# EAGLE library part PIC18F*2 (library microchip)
High-Performance, Enhanced Flash Microcontrollers with 10-Bit A/D Source: http://www.microchip.com .. 39564c.pdf
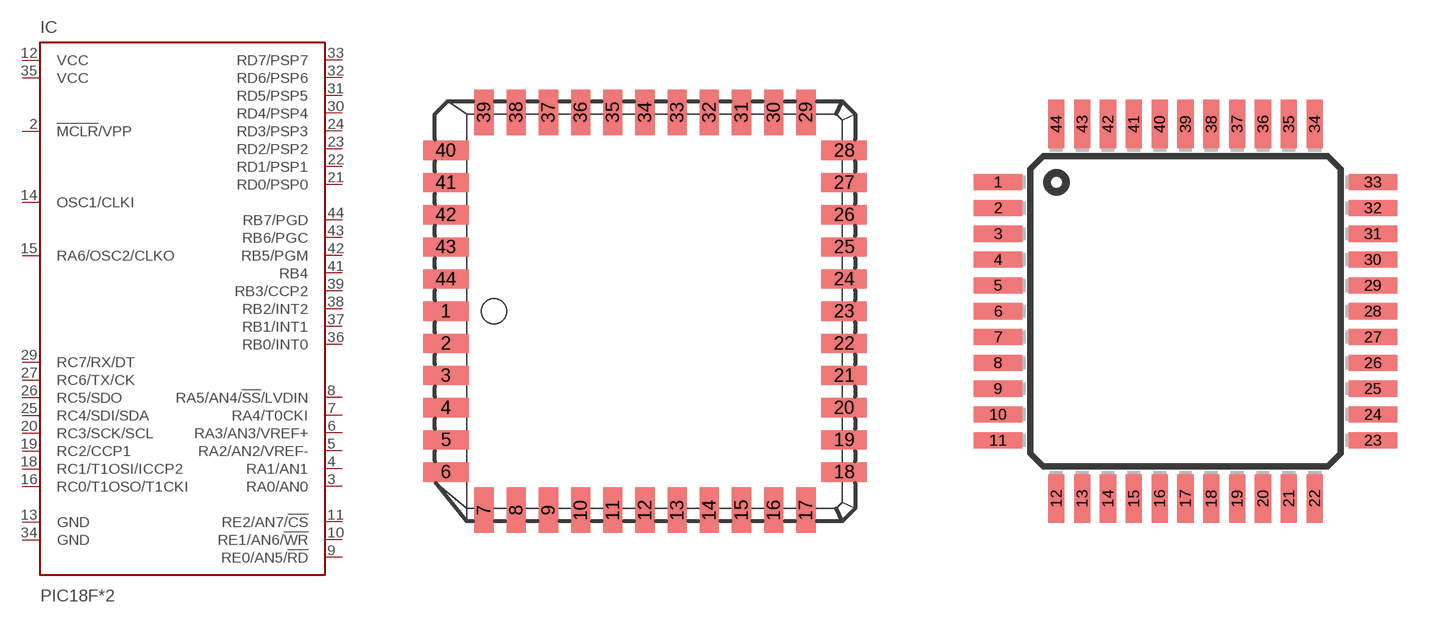
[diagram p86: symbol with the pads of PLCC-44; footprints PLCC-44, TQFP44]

Designator prefix IC

## PIC18F442L (MF: MICROCHIP; MPN: PIC18F442-E/L; OC_FARNELL: 9762175; OC_NEWARK: 72C4322), PIC18F452L (MF: MICROCHIP; MPN: PIC18F452I/L; OC_FARNELL: 9762221; OC_NEWARK: 34C8340)  [PLCC-44]
1  NC  nc
2  !MCLR!/VPP  in
3  RA0/AN0
4  RA1/AN1
5  RA2/AN2/VREF-
6  RA3/AN3/VREF+
7  RA4/T0CKI
8  RA5/AN4/!SS!/LVDIN
9  RE0/AN5/!RD
10  RE1/AN6/!WR
11  RE2/AN7/!CS
12  VCC  pwr
13  GND  pwr
14  OSC1/CLKI  in
15  RA6/OSC2/CLKO  out
16  RC0/T1OSO/T1CKI
17  NC  nc
18  RC1/T1OSI/ICCP2
19  RC2/CCP1
20  RC3/SCK/SCL
21  RD0/PSP0
22  RD1/PSP1
23  RD2/PSP2
24  RD3/PSP3
25  RC4/SDI/SDA
26  RC5/SDO
27  RC6/TX/CK
28  NC  nc
29  RC7/RX/DT
30  RD4/PSP4
31  RD5/PSP5
32  RD6/PSP6
33  RD7/PSP7
34  GND  pwr
35  VCC  pwr
36  RB0/INT0
37  RB1/INT1
38  RB2/INT2
39  RB3/CCP2
40  NC  nc
41  RB4
42  RB5/PGM
43  RB6/PGC
44  RB7/PGD

## PIC18F442PT (MF: MICROCHIP; MPN: PIC18F442-I/PT; OC_FARNELL: 1084324; OC_NEWARK: 61K3472), PIC18F452PT (MF: MICROCHIP; MPN: PIC18F452-E/PT; OC_FARNELL: 9762248; OC_NEWARK: 72C4329)  [TQFP44]
1  RC7/RX/DT
2  RD4/PSP4
3  RD5/PSP5
4  RD6/PSP6
5  RD7/PSP7
6  GND  pwr
7  VCC  pwr
8  RB0/INT0
9  RB1/INT1
10  RB2/INT2
11  RB3/CCP2
12  NC  nc
13  NC  nc
14  RB4
15  RB5/PGM
16  RB6/PGC
17  RB7/PGD
18  !MCLR!/VPP  in
19  RA0/AN0
20  RA1/AN1
21  RA2/AN2/VREF-
22  RA3/AN3/VREF+
23  RA4/T0CKI
24  RA5/AN4/!SS!/LVDIN
25  RE0/AN5/!RD
26  RE1/AN6/!WR
27  RE2/AN7/!CS
28  VCC  pwr
29  GND  pwr
30  OSC1/CLKI  in
31  RA6/OSC2/CLKO  out
32  RC0/T1OSO/T1CKI
33  NC  nc
34  NC  nc
35  RC1/T1OSI/ICCP2
36  RC2/CCP1
37  RC3/SCK/SCL
38  RD0/PSP0
39  RD1/PSP1
40  RD2/PSP2
41  RD3/PSP3
42  RC4/SDI/SDA
43  RC5/SDO
44  RC6/TX/CK

## Footprint PLCC-44 (pad centres in mm)
PLASTIC LEADED CHIP CARRIER square, package type L
smd 1.8 x 0.76: 1 -7.86,0; 2 -7.86,-1.27; 3 -7.86,-2.54; 4 -7.86,-3.81; 5 -7.86,-5.08; 6 -7.86,-6.35; 18 7.86,-6.35; 19 7.86,-5.08; 20 7.86,-3.81; 21 7.86,-2.54; 22 7.86,-1.27; 23 7.86,0; 24 7.86,1.27; 25 7.86,2.54; 26 7.86,3.81; 27 7.86,5.08; 28 7.86,6.35; 40 -7.86,6.35; 41 -7.86,5.08; 42 -7.86,3.81; 43 -7.86,2.54; 44 -7.86,1.27
smd 0.76 x 1.8: 7 -6.35,-7.86; 8 -5.08,-7.86; 9 -3.81,-7.86; 10 -2.54,-7.86; 11 -1.27,-7.86; 12 0,-7.86; 13 1.27,-7.86; 14 2.54,-7.86; 15 3.81,-7.86; 16 5.08,-7.86; 17 6.35,-7.86; 29 6.35,7.86; 30 5.08,7.86; 31 3.81,7.86; 32 2.54,7.86; 33 1.27,7.86; 34 0,7.86; 35 -1.27,7.86; 36 -2.54,7.86; 37 -3.81,7.86; 38 -5.08,7.86; 39 -6.35,7.86

## Footprint TQFP44 (pad centres in mm)
Thin Quad Flat Pack package type TQ
smd 1.5 x 0.5: 1 -5.8,4; 2 -5.8,3.2; 3 -5.8,2.4; 4 -5.8,1.6; 5 -5.8,0.8; 6 -5.8,0; 7 -5.8,-0.8; 8 -5.8,-1.6; 9 -5.8,-2.4; 10 -5.8,-3.2; 11 -5.8,-4; 23 5.8,-4; 24 5.8,-3.2; 25 5.8,-2.4; 26 5.8,-1.6; 27 5.8,-0.8; 28 5.8,0; 29 5.8,0.8; 30 5.8,1.6; 31 5.8,2.4; 32 5.8,3.2; 33 5.8,4
smd 0.5 x 1.5: 12 -4,-5.8; 13 -3.2,-5.8; 14 -2.4,-5.8; 15 -1.6,-5.8; 16 -0.8,-5.8; 17 0,-5.8; 18 0.8,-5.8; 19 1.6,-5.8; 20 2.4,-5.8; 21 3.2,-5.8; 22 4,-5.8; 34 4,5.8; 35 3.2,5.8; 36 2.4,5.8; 37 1.6,5.8; 38 0.8,5.8; 39 0,5.8; 40 -0.8,5.8; 41 -1.6,5.8; 42 -2.4,5.8; 43 -3.2,5.8; 44 -4,5.8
